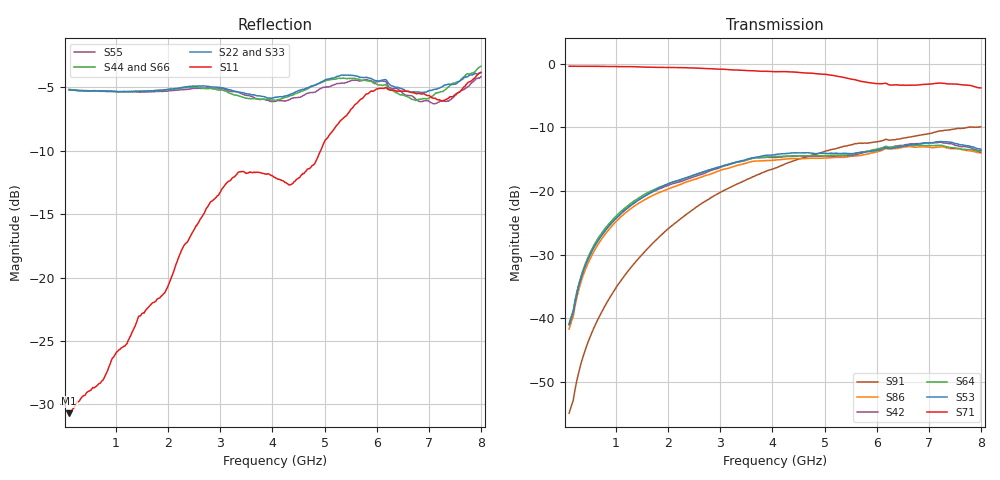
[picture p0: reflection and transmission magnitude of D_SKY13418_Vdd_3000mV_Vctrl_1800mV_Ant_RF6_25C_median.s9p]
# GHz S DB R 50
! THRU S21 mag phase subtraction.
! HALF_THRU
! EN33-165-011-v1_HALF_THRU_1 EN33-165-011-v1_HALF_THRU_2 EN33-165-011-v1_HALF_THRU_3 EN33-165-011-v1_HALF_THRU_4 EN33-165-011-v1_HALF_THRU_5 EN33-165-011-v1_HALF_THRU_6 EN33-165-011-v1_HALF_THRU_7 EN33-165-011-v1_HALF_THRU_8 EN33-165-011-v1_HALF_THRU_9
! THRU Ports: 1 2
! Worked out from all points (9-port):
!   801 points, 100 MHz to 8 GHz, reference 50 ohm
!   strongest paths, dB at 100 MHz, 2.075 GHz, 4.05 GHz, 6.025 GHz, 8 GHz:
!     S71: -0.4, -0.6, -1.2, -3.1, -3.8
!     S53: -41.0, -18.6, -14.3, -13.6, -13.4
!     S64: -40.8, -18.7, -14.6, -13.4, -13.8
!     S42: -41.0, -18.9, -14.7, -13.5, -13.6
!     S86: -41.7, -19.4, -15.1, -13.8, -14.0
!     S91: -55.0, -25.4, -16.4, -12.2, -9.9
!   lowest |S11| = -30.7 dB at 100 MHz (marker M1), VSWR 1.06, Z = 53 + j0.196 ohm
!   |S11| at or under -10 dB: start of sweep to 4.925 GHz
